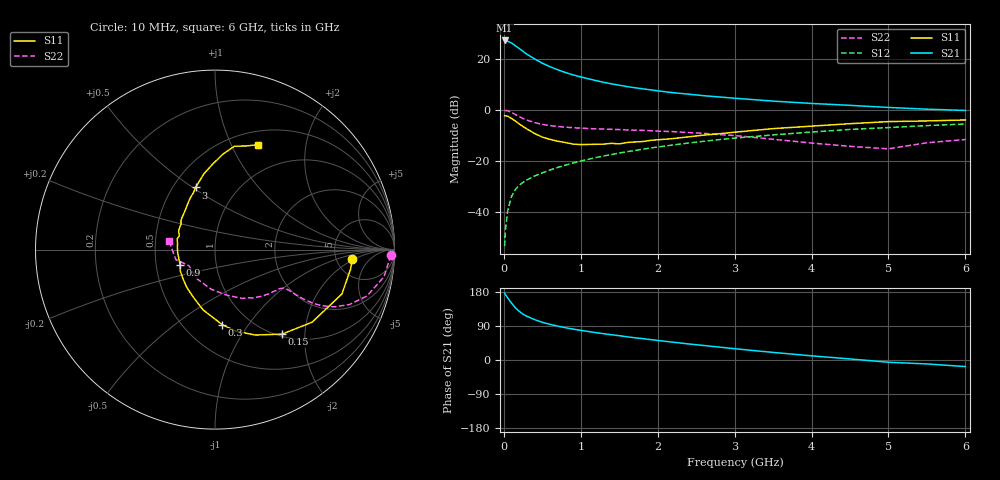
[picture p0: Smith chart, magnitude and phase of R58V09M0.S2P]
! SIEMENS Small Signal Semiconductors
! BFR183
! Si NPN RF Bipolar Junction Transistor in SOT23
! VCE = 8 V  IC = 9 mA
! Common Emitter S-Parameters:  May  1996
# GHz  S  MA  R  50
!  f  S11  S21  S12  S22
! GHz  MAG  ANG  MAG  ANG  MAG  ANG  MAG  ANG
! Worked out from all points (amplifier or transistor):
!   36 points, 10 MHz to 6 GHz, reference 50 ohm
!   highest |S21| = 27.2 dB at 10 MHz (marker M1)
!   |S21| within 3 dB of that: start of sweep to 192.8 MHz
!   unconditionally stable (mu >= 1): 853.8 MHz to 2.632 GHz
!   at 250 MHz: K = 0.58, MSG = 25.7 dB, |S12| = -28.5 dB
!   at 1.4 GHz: K = 1.05, MAG = 12.5 dB, |S12| = -17.6 dB
!   at 6 GHz: K = 0.88, MSG = 2.7 dB, |S12| = -5.6 dB
!   S11 on the Smith chart (normalised r, x): 10 MHz: 7.08, -1.78; 150 MHz: 1.04, -1.53; 300 MHz: 0.75, -0.76; 900 MHz: 0.67, -0.12; 3 GHz: 0.64, +0.51; 6 GHz: 0.65, +1.27
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0.01  0.7658 -3.9  22.95 176.4  0.0021 86.9  0.9783 -1.8
0.02  0.7636 -8.0  22.55 173.0  0.0043 84.1  0.9715 -3.8
0.05  0.749 -19.3  22.23 163.9  0.0104 78.6  0.9532 -9.2
0.1  0.6753 -36.8  20.5 150.0  0.0199 73.8  0.8851 -17.0
0.15  0.601 -51.6  18.01 137.7  0.0271 68.1  0.808 -22.3
0.2  0.5265 -64.7  15.97 128.4  0.0331 65.1  0.7356 -25.7
0.25  0.4691 -75.7  13.98 120.9  0.0377 62.7  0.6726 -27.7
0.3  0.4202 -84.5  12.33 115.2  0.042 62.5  0.6269 -28.7
0.4  0.3424 -101.2  9.954 106.6  0.0502 62.2  0.5611 -29.2
0.5  0.2902 -114.9  8.212 99.4  0.0576 62.9  0.5158 -29.1
0.6  0.2627 -126.7  7.008 94.1  0.0658 63.1  0.4885 -28.9
0.7  0.2415 -137.6  6.115 89.5  0.0737 64.1  0.4702 -28.8
0.9  0.2122 -156.5  4.843 81.5  0.0903 64.2  0.4445 -29.0
1.1  0.2088 -175.5  4.053 75.2  0.1068 64.6  0.4289 -30.3
1.3  0.2118 170.1  3.454 69.3  0.1242 63.7  0.4172 -31.8
1.6  0.2277 152.8  2.856 61.2  0.1501 62.2  0.4019 -35.3
2.2  0.272 128.1  2.165 47.0  0.2039 57.8  0.3726 -44.1
3  0.3629 107.3  1.686 29.8  0.2778 49.8  0.3124 -60.6
3.5  0.4264 98.4  1.479 20.0  0.321 43.7  0.2639 -75.0
4.5  0.5332 85.3  1.221 2.8  0.4117 31.9  0.1915 -120.6
5.5  0.604 73.0  1.028 -10.4  0.4892 20.4  0.2252 -165.7
6  0.6313 67.8  0.97 -17.3  0.526 12.8  0.2604 169.6
